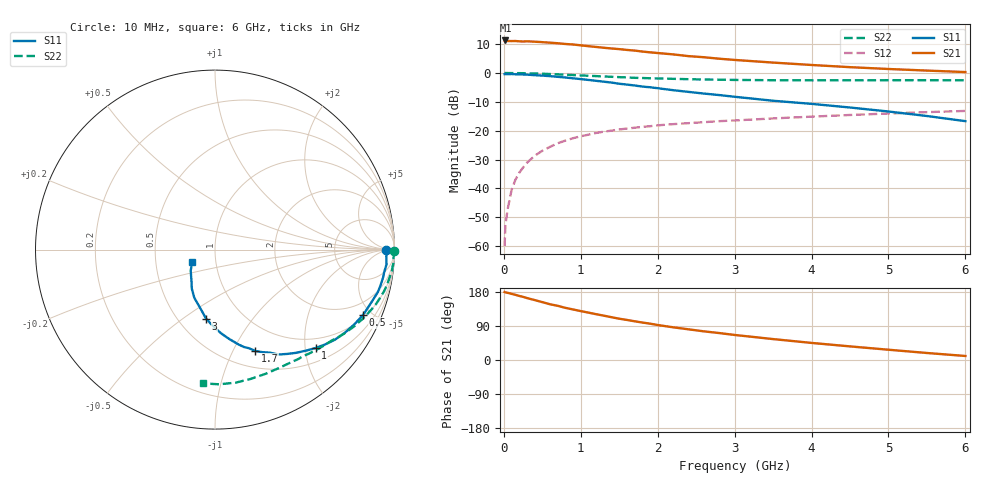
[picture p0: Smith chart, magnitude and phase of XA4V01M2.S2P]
! SIEMENS Discrete & RF Semiconductors
! BFY180
! Si NPN RF Bipolar Junction Transistor in MICRO-X
! VCE = 4 V  IC = 1.2 mA
! Common Emitter S-Parameters:  May  1997
# GHz  S  MA  R  50
!  f  S11  S21  S12  S22
! GHz  MAG  ANG  MAG  ANG  MAG  ANG  MAG  ANG
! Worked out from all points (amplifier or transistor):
!   36 points, 10 MHz to 6 GHz, reference 50 ohm
!   highest |S21| = 11.3 dB at 20 MHz (marker M1)
!   |S21| within 3 dB of that: start of sweep to 1.499 GHz
!   unconditionally stable (mu >= 1): 3.64 GHz to end of sweep
!   at 250 MHz: K = 0.08, MSG = 21.8 dB, |S12| = -32.8 dB
!   at 1.4 GHz: K = 0.53, MSG = 14.2 dB, |S12| = -20.0 dB
!   at 6 GHz: K = 1.06, MAG = 5.2 dB, |S12| = -13.1 dB
!   S11 on the Smith chart (normalised r, x): 10 MHz: 43, -5; 500 MHz: 1.14, -4.47; 1 GHz: 0.78, -2.22; 1.7 GHz: 0.69, -1.23; 3 GHz: 0.68, -0.61; 6 GHz: 0.77, -0.11
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0.01  0.9553 -0.3  3.566 179.4  0.001 88.4  0.997 -0.3
0.02  0.9589 -0.9  3.662 178.5  0.0023 93.5  0.9999 -0.7
0.05  0.9551 -2.3  3.582 177.3  0.0044 84.8  0.9977 -1.4
0.1  0.9592 -4.9  3.572 174.6  0.0093 91.0  0.9953 -2.8
0.15  0.9504 -7.8  3.58 172.0  0.0141 86.4  0.997 -4.2
0.3  0.9375 -14.7  3.542 163.5  0.0278 79.7  0.9872 -8.3
0.5  0.9019 -23.8  3.422 152.7  0.0449 73.8  0.9707 -13.7
0.6  0.8811 -28.2  3.352 147.1  0.0526 70.8  0.9594 -16.1
0.7  0.8587 -32.7  3.279 143.0  0.0606 67.7  0.9475 -18.6
0.8  0.8353 -37.0  3.182 137.6  0.0675 65.1  0.9339 -20.9
1  0.7838 -44.4  3.012 129.0  0.0802 59.8  0.9079 -25.3
1.1  0.7582 -47.9  2.914 125.0  0.0854 57.7  0.895 -27.2
1.5  0.6511 -61.9  2.592 109.0  0.1051 49.9  0.8477 -34.6
1.7  0.6079 -68.3  2.447 102.2  0.1126 47.0  0.8249 -37.8
2  0.5452 -76.0  2.218 92.3  0.1239 43.0  0.8053 -42.2
2.2  0.504 -81.0  2.101 86.3  0.13 40.5  0.7919 -45.2
2.6  0.4402 -89.6  1.876 75.6  0.1406 36.7  0.7711 -50.4
3  0.3874 -97.4  1.684 66.1  0.1506 33.1  0.7585 -55.5
3.5  0.3306 -105.1  1.515 55.2  0.1633 29.4  0.7499 -61.7
4.5  0.2525 -120.8  1.262 35.9  0.1874 21.9  0.7475 -74.6
5.5  0.1799 -138.8  1.101 18.5  0.2099 14.4  0.7507 -88.3
6  0.1465 -150.9  1.038 10.6  0.2202 10.1  0.7486 -95.3
